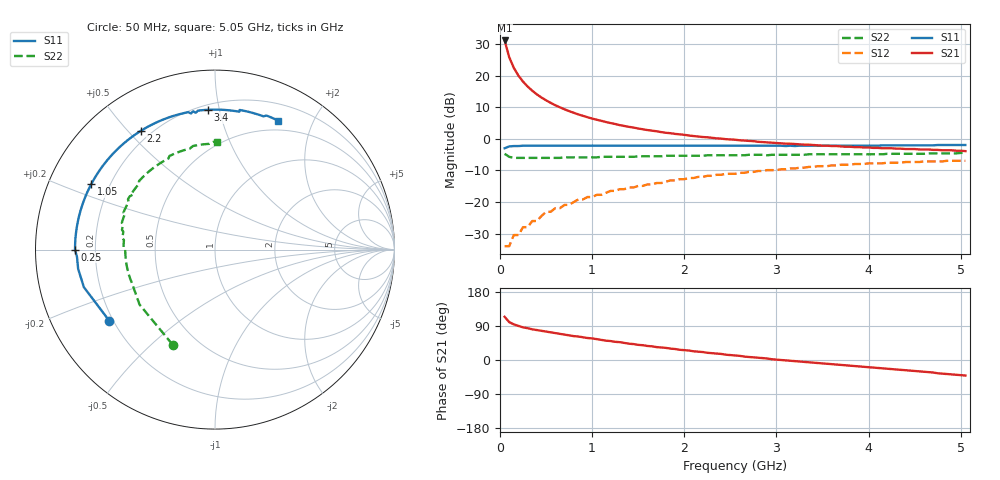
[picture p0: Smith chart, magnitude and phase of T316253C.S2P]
!AT-31625
!S-PARAMETERS at Vce=3.0 V  Ic=150 mA.  LAST UPDATED 08-05-96
# ghz s ma r 50
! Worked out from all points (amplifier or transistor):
!   101 points, 50 MHz to 5.05 GHz, reference 50 ohm
!   highest |S21| = 31.2 dB at 50 MHz (marker M1)
!   |S21| within 3 dB of that: start of sweep to 78.29 MHz
!   unconditionally stable (mu >= 1): 390.8 MHz to 426 MHz; 524.8 MHz to 1.699 GHz; 1.701 GHz to 1.814 GHz
!   at 850 MHz: K = 1.01, MAG = 12.7 dB, |S12| = -19.2 dB
!   at 2.55 GHz: K = 0.97, MSG = 5.4 dB, |S12| = -11.1 dB
!   at 5.05 GHz: K = 0.96, MSG = 1.5 dB, |S12| = -6.9 dB
!   S11 on the Smith chart (normalised r, x): 50 MHz: 0.18, -0.30; 250 MHz: 0.12, -0.00; 1.05 GHz: 0.13, +0.25; 2.2 GHz: 0.16, +0.54; 3.4 GHz: 0.23, +0.92; 5.05 GHz: 0.38, +1.53
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0.05  0.71 -146.0  36.2 114.0  0.02 41.0  0.58 -114.0
0.1  0.76 -164.0  19.66 100.0  0.02 42.0  0.52 -144.0
0.15  0.77 -172.0  13.31 94.0  0.03 48.0  0.5 -156.0
0.2  0.77 -177.0  10.05 90.0  0.03 52.0  0.5 -163.0
0.25  0.78 -180.0  8.07 86.0  0.04 56.0  0.5 -167.0
0.3  0.78 177.0  6.74 84.0  0.04 59.0  0.5 -170.0
0.35  0.78 175.0  5.79 81.0  0.05 60.0  0.5 -172.0
0.4  0.78 173.0  5.07 79.0  0.05 62.0  0.5 -174.0
0.45  0.78 171.0  4.52 77.0  0.06 62.0  0.5 -175.0
0.55  0.78 167.0  3.72 73.0  0.07 63.0  0.5 -178.0
0.65  0.78 164.0  3.16 69.0  0.08 64.0  0.5 -180.0
0.75  0.78 161.0  2.75 65.0  0.09 63.0  0.51 178.0
0.9  0.78 157.0  2.32 60.0  0.11 62.0  0.51 176.0
1.05  0.78 152.0  2.01 55.0  0.13 60.0  0.51 174.0
1.15  0.78 149.0  1.85 51.0  0.14 59.0  0.52 173.0
1.4  0.78 143.0  1.55 43.0  0.17 55.0  0.52 169.0
1.75  0.78 134.0  1.28 33.0  0.2 50.0  0.53 165.0
2.2  0.78 122.0  1.07 21.0  0.25 42.0  0.54 158.0
2.55  0.78 113.0  0.97 12.0  0.28 35.0  0.55 153.0
3.4  0.78 93.0  0.8 -7.0  0.36 20.0  0.57 137.0
4.25  0.79 78.0  0.71 -24.0  0.42 1.0  0.58 114.0
5.05  0.8 64.0  0.64 -41.0  0.45 -15.0  0.6 89.0
